(* Logix 5000 Controller export Example_PLC; controller Example_PLC 1769-L32E rev 19.11; software revision 19.01 *)

TASK MainTask (continuous, watchdog 500 ms) : MainProgram

MODULES
   Controller : 1769-L32E (CompactLogixL32EController 0, rev 19.11)
      LocalENB : 1769-L32E Ethernet Port (CompactLogixL32Ethernet 1, Ethernet 192.168.0.3, rev 19.11)
         AKD_1 : ETHERNET-MODULE (Ethernet 10.8.46.174, rev 1.1, Output RPI 40 ms)
      Local : CompactBus (CompactVirtualAdapter 3, rev 19.11)
END_MODULES

TYPE AKD_Axis :   // Axis Data:
STRUCT
   Control : AKD_Control;   // Control bits to send to the drive
   Status : AKD_Status;   // Status bits received from the drive
   Input : AB:ETHERNET_MODULE_SINT_64Bytes:I:0;   // Data from the drive
   Output : AB:ETHERNET_MODULE_SINT_64Bytes:O:0;   // Data to the drive
   ResponseMsgType : SINT;   // Response type contained in latest IO response from drive. Used to check for errors
   CommandTimeout : INT;   // Time to allow for command response from drive. Dependent on scan rate and communicaiton rate
   PositionFeedback : DINT;   // Actual Position Value
   VelocityFeedback : DINT;   // Actual Velocity Value
END_STRUCT
END_TYPE

TYPE AKD_Control :   // Send Explicit Message
STRUCT
   Load_Data_Start_Profile : BOOL;   // Load Command Data / Start Profile Move
   Start_Block : BOOL;   // Execute Command block or block chain
   Incremental : BOOL;   // Incremental Position (0=Absolute, 1=Incremental)
   Direction : BOOL;   // Direction in Velocity Mode (0=Reverse, 1=Forward)
   Smooth_Stop : BOOL;   // Smooth / Controlled Stop w/ Deceleration
   Hard_Stop : BOOL;   // Hard / Immediate Stop
   Reg_Arm : BOOL;   // Arm the Registration Input
   Enable : BOOL;   // Enable Output
END_STRUCT
END_TYPE

TYPE AKD_Status :   // All connections to the drive ethernet module are established and data is successfully transferring.
STRUCT
   Profile_In_Progress : BOOL;   // Profile Move In Progress
   Block_In_Execution : BOOL;   // Block In Execution
   On_Target_Position : BOOL;   // On Target Position (1=Current Position Equals Last Target Position)
   General_Fault : BOOL;   // General Fault
   Current_Direction : BOOL;   // Current Motor Direction (0=Reverse, 1=Forward)
   Home_Level : BOOL;   // Level of Home Input
   Reg_Level : BOOL;   // Level of Registration Input
   Enable : BOOL;   // State of Enable Output
   Fault_Input_Fault : BOOL;   // Fault Input Active
   Fwd_Limit : BOOL;   // Forward Input Active
   Rev_Limit : BOOL;   // Reverse Input Active
   Positive_Limit : BOOL;   // Positive Software Limit Exceeded
   Negative_Limit : BOOL;   // Negative Software Limit Exceeded
   FE_Fault : BOOL;   // Following Error Fault
   Block_Fault : BOOL;   // Block Execution Fault
   Load_Complete : BOOL;   // Command Message Successfully Loaded
END_STRUCT
END_TYPE

TYPE Motion_Task :
STRUCT
   Accel : LINT;   // MT.ACC Acceleration
   ControlWord : DINT;   // MT.CNTL
   Decel : LINT;   // MT.DEC
   Delay : INT;   // MT.TNEXT Delay before executing next task
   NextNum : SINT;   // MT.TNEXT Number of next task to execute
   Position : LINT;   // MT.P Target Position
   Num : SINT;   // MT.NUM Number of this task in the table
   Velocity : LINT;   // MT.V Target Velocity
   Set : SINT;   // Used to command a set of the MT. Should always equal 1
END_STRUCT
END_TYPE

ADD_ON_INSTRUCTION AKD_Disable   (* revision 2.1, ExecutePrescan, ExecuteEnableInFalse *)
// Disable Drive
// Revision note:
// Don't error if Command_Timeout preset is 0
VAR_OUTPUT
   DN : BOOL; {access Read Only, visible}   // Command Successful
   ER : BOOL; {access Read Only, visible}   // Error
END_VAR
VAR_IN_OUT
   Axis : AKD_Axis; {required}
END_VAR
VAR
   Command_Timeout : TIMER := (PRE := 200);   // Timeout Timer
END_VAR

ROUTINE EnableInFalse   (* ladder *)
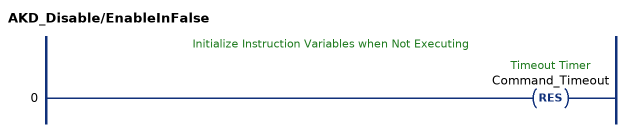
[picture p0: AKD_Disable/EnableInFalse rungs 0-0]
   // Initialize Instruction Variables when Not Executing
   0: RES(Command_Timeout);
END_ROUTINE

ROUTINE Logic   (* ladder *)
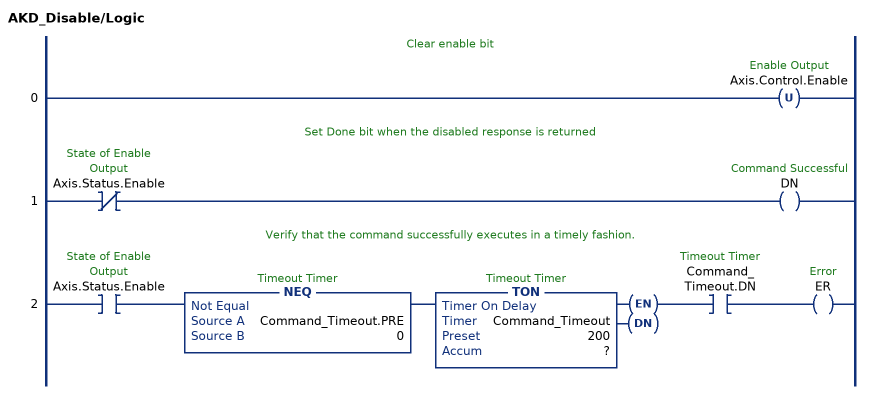
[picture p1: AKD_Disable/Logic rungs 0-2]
   // Clear enable bit
   0: OTU(Axis.Control.Enable);
   // Set Done bit when the disabled response is returned
   1: XIO(Axis.Status.Enable)OTE(DN);
   // Verify that the command successfully executes in a timely fashion.
   2: XIC(Axis.Status.Enable)NEQ(Command_Timeout.PRE,0)TON(Command_Timeout,?,?)XIC(Command_Timeout.DN)OTE(ER);
END_ROUTINE

ROUTINE Prescan   (* ladder *)
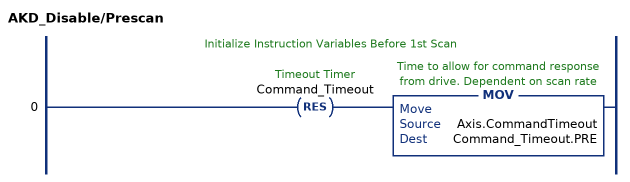
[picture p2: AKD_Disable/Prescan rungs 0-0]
   // Initialize Instruction Variables Before 1st Scan
   0: RES(Command_Timeout)MOV(Axis.CommandTimeout,Command_Timeout.PRE);
END_ROUTINE
END_ADD_ON_INSTRUCTION

ADD_ON_INSTRUCTION AKD_Drive   (* revision 2.0, ExecutePrescan *)
// Drive Communication
VAR_IN_OUT
   Axis_Input : AB:ETHERNET_MODULE_SINT_64Bytes:I:0; {required}
   Axis_Output : AB:ETHERNET_MODULE_SINT_64Bytes:O:0; {required}
   Axis_Internal : AKD_Axis; {required}
END_VAR
VAR
   Command_Bytes : SINT[8];
   Response_Bytes : SINT[8];
END_VAR

ROUTINE Logic   (* ladder *)
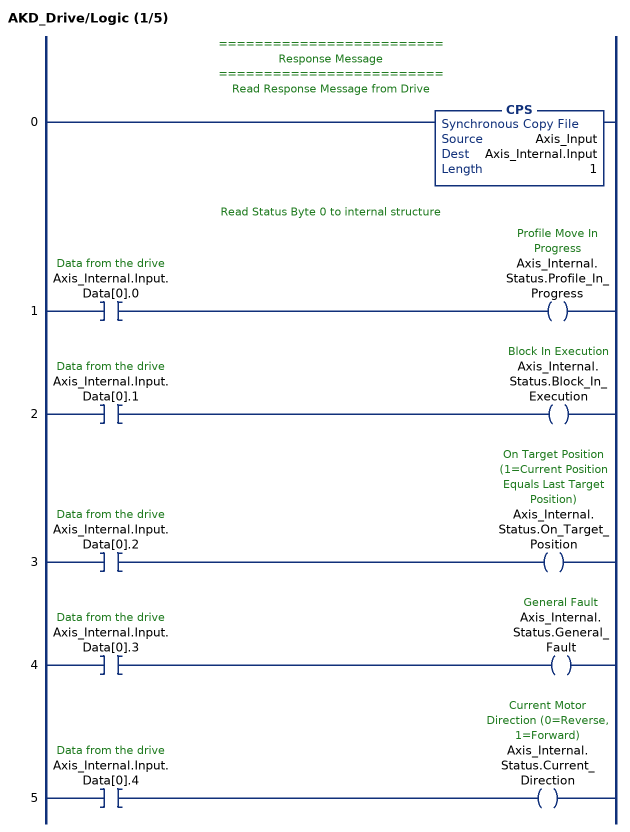
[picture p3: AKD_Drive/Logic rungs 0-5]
   // =========================
   // Response Message
   // =========================
   // Read Response Message from Drive
   0: CPS(Axis_Input,Axis_Internal.Input,1);
   // Read Status Byte 0 to internal structure
   1: XIC(Axis_Internal.Input.Data[0].0)OTE(Axis_Internal.Status.Profile_In_Progress);
   2: XIC(Axis_Internal.Input.Data[0].1)OTE(Axis_Internal.Status.Block_In_Execution);
   3: XIC(Axis_Internal.Input.Data[0].2)OTE(Axis_Internal.Status.On_Target_Position);
   4: XIC(Axis_Internal.Input.Data[0].3)OTE(Axis_Internal.Status.General_Fault);
   5: XIC(Axis_Internal.Input.Data[0].4)OTE(Axis_Internal.Status.Current_Direction);
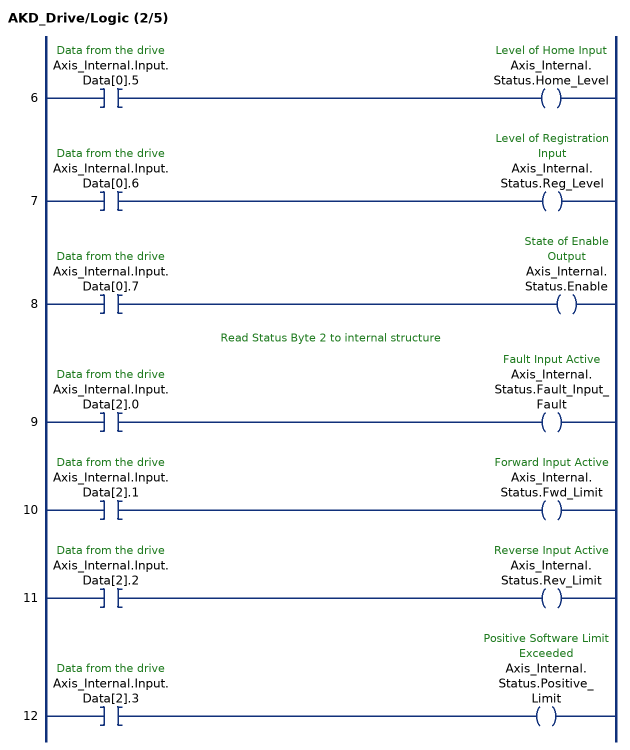
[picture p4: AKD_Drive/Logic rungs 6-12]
   6: XIC(Axis_Internal.Input.Data[0].5)OTE(Axis_Internal.Status.Home_Level);
   7: XIC(Axis_Internal.Input.Data[0].6)OTE(Axis_Internal.Status.Reg_Level);
   8: XIC(Axis_Internal.Input.Data[0].7)OTE(Axis_Internal.Status.Enable);
   // Read Status Byte 2 to internal structure
   9: XIC(Axis_Internal.Input.Data[2].0)OTE(Axis_Internal.Status.Fault_Input_Fault);
   10: XIC(Axis_Internal.Input.Data[2].1)OTE(Axis_Internal.Status.Fwd_Limit);
   11: XIC(Axis_Internal.Input.Data[2].2)OTE(Axis_Internal.Status.Rev_Limit);
   12: XIC(Axis_Internal.Input.Data[2].3)OTE(Axis_Internal.Status.Positive_Limit);
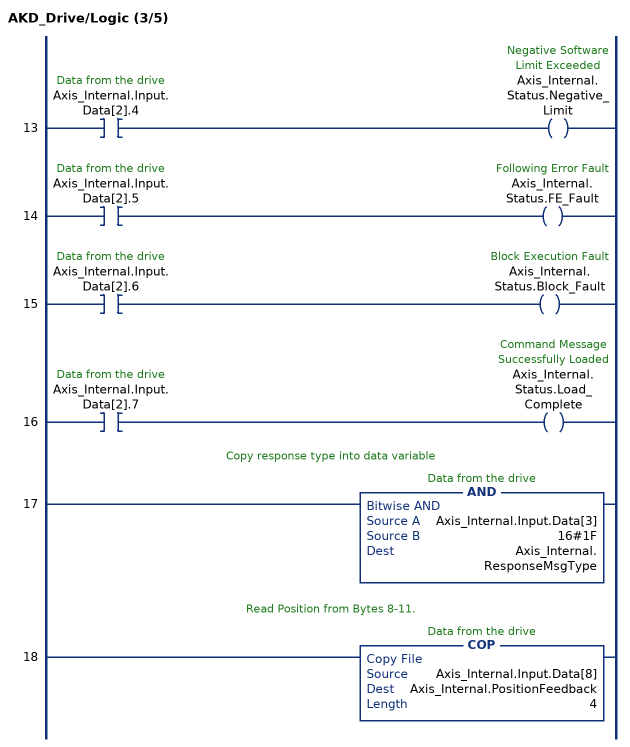
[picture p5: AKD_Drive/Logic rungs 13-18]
   13: XIC(Axis_Internal.Input.Data[2].4)OTE(Axis_Internal.Status.Negative_Limit);
   14: XIC(Axis_Internal.Input.Data[2].5)OTE(Axis_Internal.Status.FE_Fault);
   15: XIC(Axis_Internal.Input.Data[2].6)OTE(Axis_Internal.Status.Block_Fault);
   16: XIC(Axis_Internal.Input.Data[2].7)OTE(Axis_Internal.Status.Load_Complete);
   // Copy response type into data variable
   17: AND(Axis_Internal.Input.Data[3],16#1F,Axis_Internal.ResponseMsgType);
   // Read Position from Bytes 8-11.
   18: COP(Axis_Internal.Input.Data[8],Axis_Internal.PositionFeedback,4);
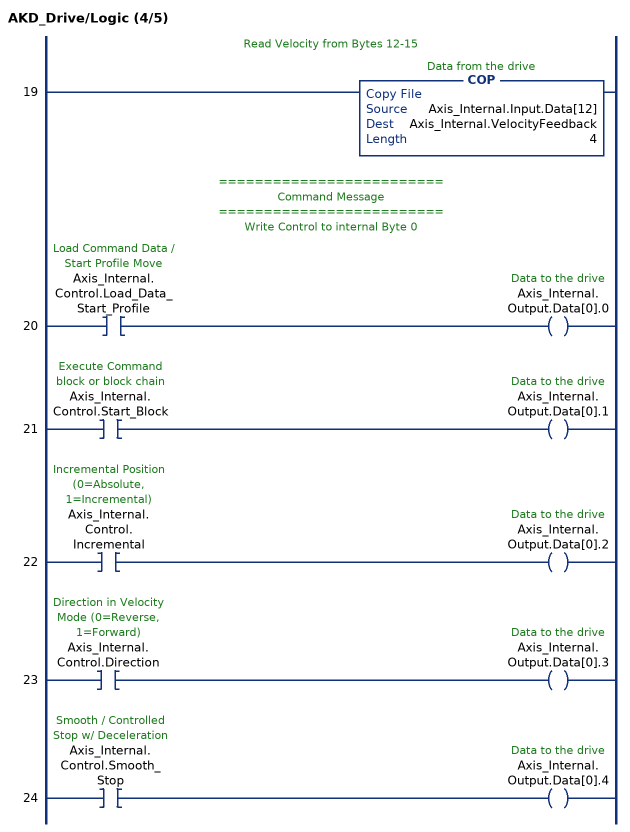
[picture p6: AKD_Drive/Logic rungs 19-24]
   // Read Velocity from Bytes 12-15
   19: COP(Axis_Internal.Input.Data[12],Axis_Internal.VelocityFeedback,4);
   // =========================
   // Command Message
   // =========================
   // Write Control to internal Byte 0
   20: XIC(Axis_Internal.Control.Load_Data_Start_Profile)OTE(Axis_Internal.Output.Data[0].0);
   21: XIC(Axis_Internal.Control.Start_Block)OTE(Axis_Internal.Output.Data[0].1);
   22: XIC(Axis_Internal.Control.Incremental)OTE(Axis_Internal.Output.Data[0].2);
   23: XIC(Axis_Internal.Control.Direction)OTE(Axis_Internal.Output.Data[0].3);
   24: XIC(Axis_Internal.Control.Smooth_Stop)OTE(Axis_Internal.Output.Data[0].4);
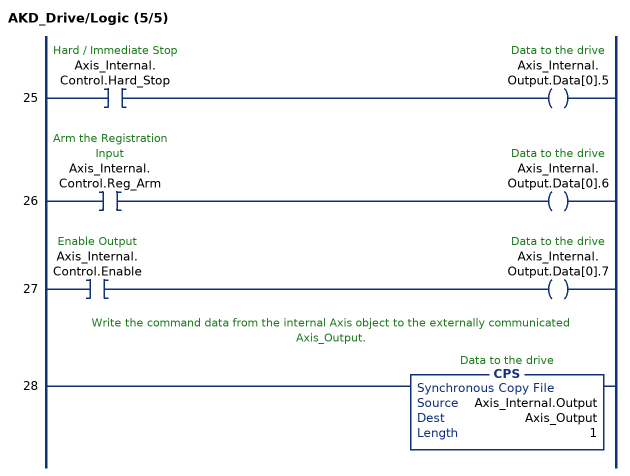
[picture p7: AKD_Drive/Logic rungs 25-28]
   25: XIC(Axis_Internal.Control.Hard_Stop)OTE(Axis_Internal.Output.Data[0].5);
   26: XIC(Axis_Internal.Control.Reg_Arm)OTE(Axis_Internal.Output.Data[0].6);
   27: XIC(Axis_Internal.Control.Enable)OTE(Axis_Internal.Output.Data[0].7);
   // Write the command data from the internal Axis object to the externally communicated Axis_Output.
   28: CPS(Axis_Internal.Output,Axis_Output,1);
END_ROUTINE

ROUTINE Prescan   (* ladder *)
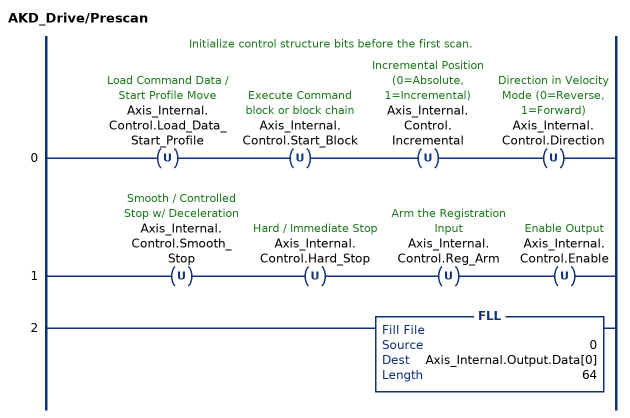
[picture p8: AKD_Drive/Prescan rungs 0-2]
   // Initialize control structure bits before the first scan.
   0: OTU(Axis_Internal.Control.Load_Data_Start_Profile)OTU(Axis_Internal.Control.Start_Block)OTU(Axis_Internal.Control.Incremental)OTU(Axis_Internal.Control.Direction);
   1: OTU(Axis_Internal.Control.Smooth_Stop)OTU(Axis_Internal.Control.Hard_Stop)OTU(Axis_Internal.Control.Reg_Arm)OTU(Axis_Internal.Control.Enable);
   2: FLL(0,Axis_Internal.Output.Data[0],64);
END_ROUTINE
END_ADD_ON_INSTRUCTION

ADD_ON_INSTRUCTION AKD_Enable   (* revision 2.0, ExecutePrescan, ExecuteEnableInFalse *)
// Enables Drive
VAR_OUTPUT
   DN : BOOL; {access Read Only, visible}   // Command Successful
   ER : BOOL; {access Read Only, visible}   // Error
END_VAR
VAR_IN_OUT
   Axis : AKD_Axis; {required}
END_VAR
VAR
   Command_Timeout : TIMER := (PRE := 2000);   // Timeout Timer
   Transition : BOOL;   // Marker to transition enable bit if required.
   Transition_Complete : BOOL;   // Flag to indicate that no further transistion is required.
END_VAR

ROUTINE EnableInFalse   (* ladder *)
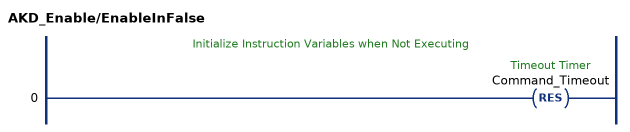
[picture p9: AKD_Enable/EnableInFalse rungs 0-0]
   // Initialize Instruction Variables when Not Executing
   0: RES(Command_Timeout);
END_ROUTINE

ROUTINE Logic   (* ladder *)
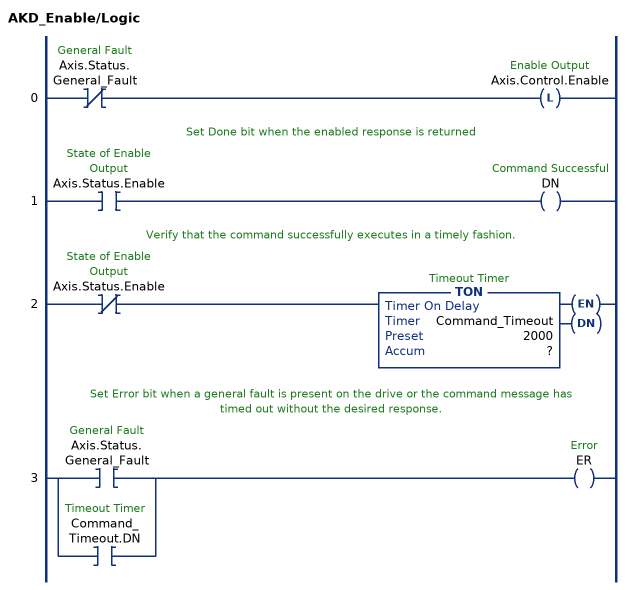
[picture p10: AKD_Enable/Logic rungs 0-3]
   0: XIO(Axis.Status.General_Fault)OTL(Axis.Control.Enable);
   // Set Done bit when the enabled response is returned
   1: XIC(Axis.Status.Enable)OTE(DN);
   // Verify that the command successfully executes in a timely fashion.
   2: XIO(Axis.Status.Enable)TON(Command_Timeout,?,?);
   // Set Error bit when a general fault is present on the drive or the command message has timed out without the desired response.
   3: [XIC(Axis.Status.General_Fault) ,XIC(Command_Timeout.DN) ]OTE(ER);
END_ROUTINE

ROUTINE Prescan   (* ladder *)
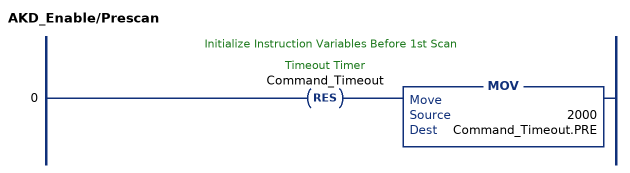
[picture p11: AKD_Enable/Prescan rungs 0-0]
   // Initialize Instruction Variables Before 1st Scan
   0: RES(Command_Timeout)MOV(2000,Command_Timeout.PRE);
END_ROUTINE
END_ADD_ON_INSTRUCTION

ADD_ON_INSTRUCTION AKD_Set_Accel   (* revision 2.1, ExecutePrescan, ExecuteEnableInFalse *)
// Set Drive Acceleration
// Revision note:
// Don't error if Command_Timeout preset is 0
VAR_OUTPUT
   DN : BOOL; {access Read Only, visible}   // Command Successful
   ER : BOOL; {access Read Only, visible}   // Error
END_VAR
VAR_IN_OUT
   Axis : AKD_Axis; {required}
END_VAR
VAR_INPUT
   Accel : DINT; {required}   // Acceleration
END_VAR
VAR
   Response_Bytes : SINT[8];
   Accel_Internal : DINT;   // Scaled Accel Value for Drive
   Command_Timeout : TIMER := (PRE := 100);   // Timeout Timer
   Command_Message_Type : SINT;   // Command Message Type
   Command_Axis_Number : SINT;   // Command Axis Number
   Response_Message_Type : SINT;   // Response Message Type
   Response_Axis_Number : SINT;   // Response Axis Number
   Command_Bytes : SINT[8];
   OS_LoadStart : BOOL;
   Step : SINT;
END_VAR

ROUTINE EnableInFalse   (* ladder *)
// EnableIn_False
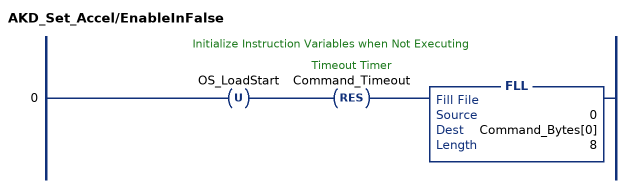
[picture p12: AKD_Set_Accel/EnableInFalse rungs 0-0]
   // Initialize Instruction Variables when Not Executing
   0: OTU(OS_LoadStart)RES(Command_Timeout)FLL(0,Command_Bytes[0],8);
END_ROUTINE

ROUTINE Logic   (* ladder *)
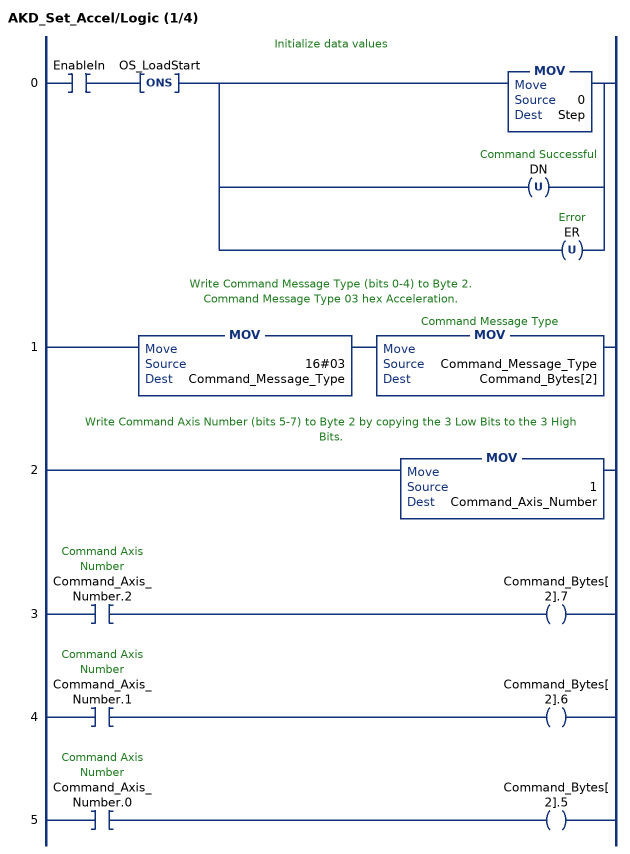
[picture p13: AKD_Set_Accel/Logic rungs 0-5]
   // Initialize data values
   0: XIC(EnableIn)ONS(OS_LoadStart)[MOV(0,Step) ,OTU(DN) ,OTU(ER) ];
   // Write Command Message Type (bits 0-4) to Byte 2.
   // Command Message Type 03 hex Acceleration.
   1: MOV(16#03,Command_Message_Type)MOV(Command_Message_Type,Command_Bytes[2]);
   // Write Command Axis Number (bits 5-7) to Byte 2 by copying the 3 Low Bits to the 3 High Bits.
   2: MOV(1,Command_Axis_Number);
   3: XIC(Command_Axis_Number.2)OTE(Command_Bytes[2].7);
   4: XIC(Command_Axis_Number.1)OTE(Command_Bytes[2].6);
   5: XIC(Command_Axis_Number.0)OTE(Command_Bytes[2].5);
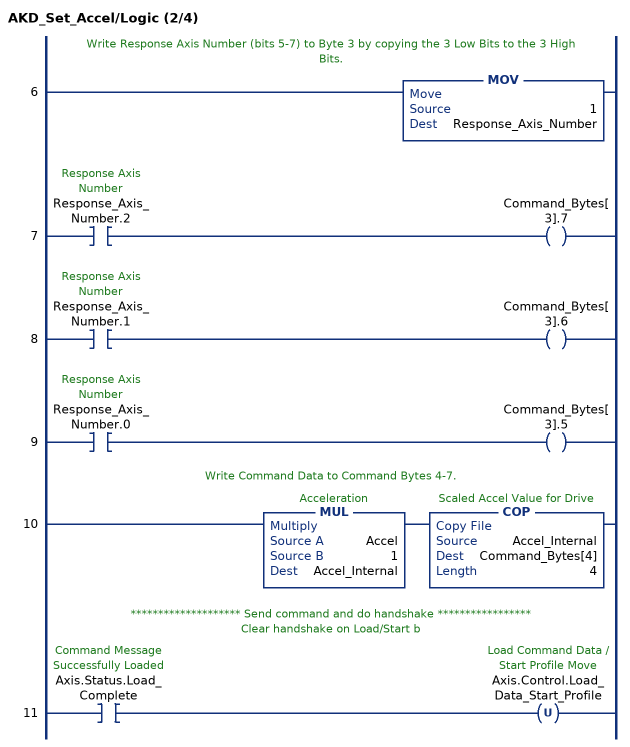
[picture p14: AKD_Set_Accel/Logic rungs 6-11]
   // Write Response Axis Number (bits 5-7) to Byte 3 by copying the 3 Low Bits to the 3 High Bits.
   6: MOV(1,Response_Axis_Number);
   7: XIC(Response_Axis_Number.2)OTE(Command_Bytes[3].7);
   8: XIC(Response_Axis_Number.1)OTE(Command_Bytes[3].6);
   9: XIC(Response_Axis_Number.0)OTE(Command_Bytes[3].5);
   // Write Command Data to Command Bytes 4-7.
   10: MUL(Accel,1,Accel_Internal)COP(Accel_Internal,Command_Bytes[4],4);
   // ******************** Send command and do handshake *****************
   // Clear handshake on Load/Start b
   11: XIC(Axis.Status.Load_Complete)OTU(Axis.Control.Load_Data_Start_Profile);
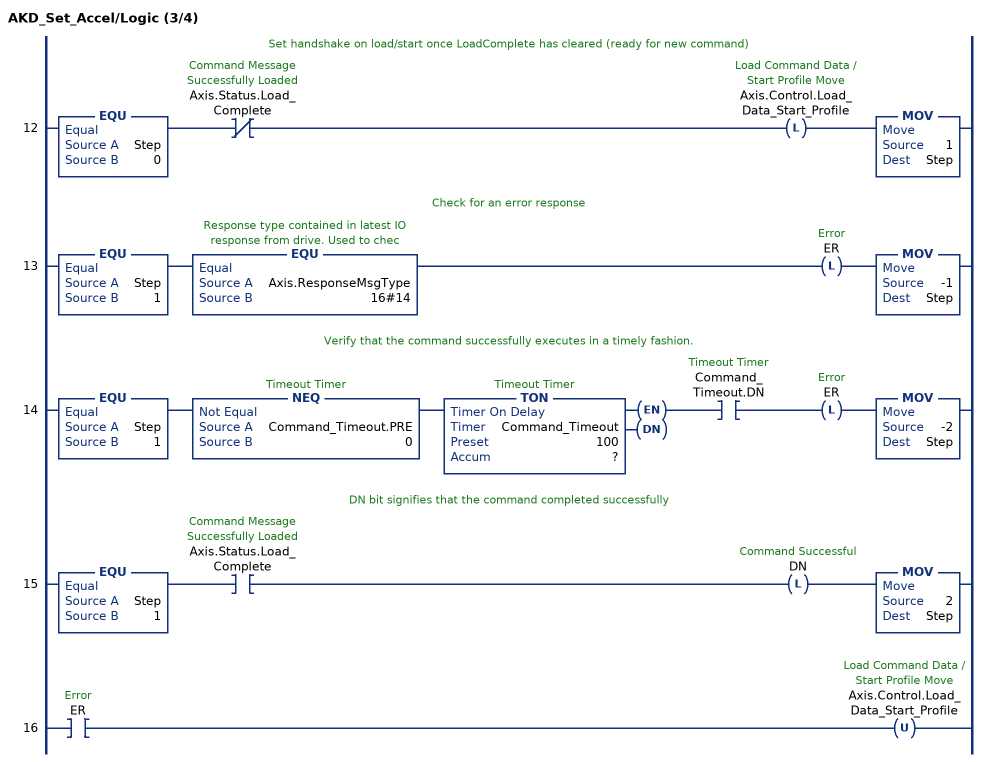
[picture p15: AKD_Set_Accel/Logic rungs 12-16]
   // Set handshake on load/start once LoadComplete has cleared (ready for new command)
   12: EQU(Step,0)XIO(Axis.Status.Load_Complete)OTL(Axis.Control.Load_Data_Start_Profile)MOV(1,Step);
   // Check for an error response
   13: EQU(Step,1)EQU(Axis.ResponseMsgType,16#14)OTL(ER)MOV(-1,Step);
   // Verify that the command successfully executes in a timely fashion.
   14: EQU(Step,1)NEQ(Command_Timeout.PRE,0)TON(Command_Timeout,?,?)XIC(Command_Timeout.DN)OTL(ER)MOV(-2,Step);
   // DN bit signifies that the command completed successfully
   15: EQU(Step,1)XIC(Axis.Status.Load_Complete)OTL(DN)MOV(2,Step);
   16: XIC(ER)OTU(Axis.Control.Load_Data_Start_Profile);
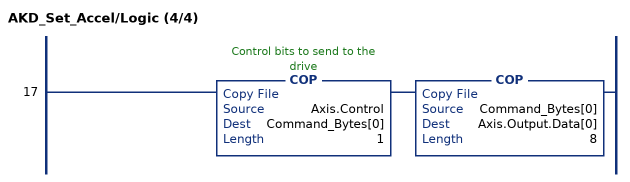
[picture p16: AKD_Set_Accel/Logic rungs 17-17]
   17: COP(Axis.Control,Command_Bytes[0],1)COP(Command_Bytes[0],Axis.Output.Data[0],8);
END_ROUTINE

ROUTINE Prescan   (* ladder *)
// Prescan
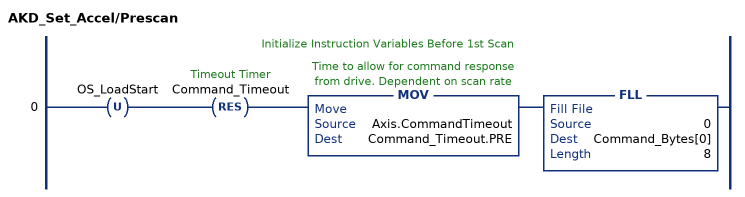
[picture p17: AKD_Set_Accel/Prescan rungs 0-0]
   // Initialize Instruction Variables Before 1st Scan
   0: OTU(OS_LoadStart)RES(Command_Timeout)MOV(Axis.CommandTimeout,Command_Timeout.PRE)FLL(0,Command_Bytes[0],8);
END_ROUTINE
END_ADD_ON_INSTRUCTION
